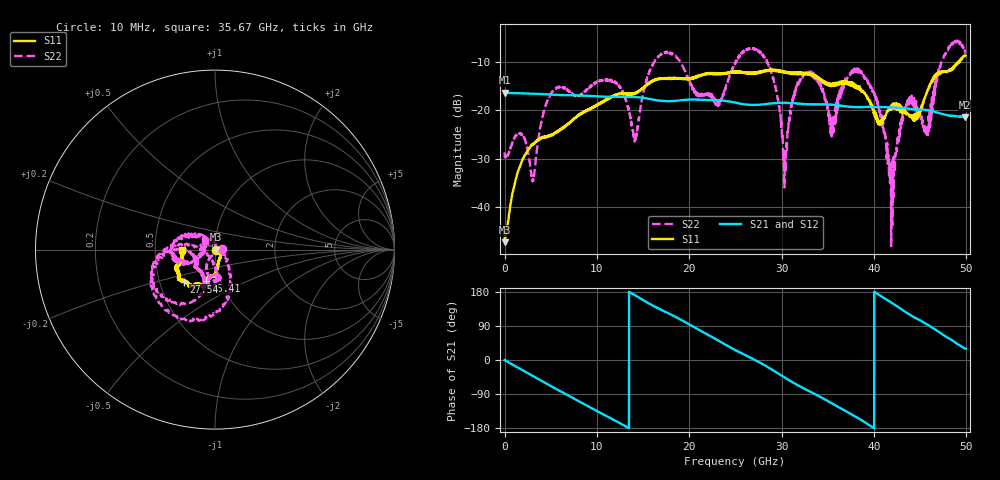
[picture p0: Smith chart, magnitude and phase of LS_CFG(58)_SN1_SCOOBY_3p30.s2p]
!Keysight Technologies,N5245B,MY58422026,A.13.80.08
!Date: Thursday, March 19, 2020 23:45:07
!Correction: S11(Full 2 Port(1,2))
!S21(Full 2 Port(1,2))
!S12(Full 2 Port(1,2))
!S22(Full 2 Port(1,2))
!S2P File: Measurements: S11, S21, S12, S22:
# Hz S DB R 50.0
!freq dBS11 angS11 dBS21 angS21 dBS12 angS12 dBS22 angS22
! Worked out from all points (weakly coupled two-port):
!   4991 points, 10 MHz to 49.91 GHz, reference 50 ohm
!   highest |S21| = -16.38 dB at 10 MHz (marker M1); lowest = -21.4 dB at 49.82 GHz (marker M2)
!   lowest |S11| = -47.2 dB at 30 MHz (marker M3), VSWR 1.01, Z = 50.4 - j0.0242 ohm
!   |S11| at or under -10 dB: start of sweep to 49.13 GHz; 49.1623 GHz to 49.22728 GHz (64.98 MHz wide, 0.132 % of centre)
!   |S22| runs from -48.0 to -5.6 dB; largest |S21 - S12| = 0.0015
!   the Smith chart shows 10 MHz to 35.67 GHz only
!   S11 on the Smith chart (normalised r, x): 10 MHz: 1.01, -0.01; 15.41 GHz: 0.85, -0.31; 27.54 GHz: 0.66, -0.25; 35.67 GHz: 0.69, -0.01
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1e7  -45.23 -31.8  -16.38 -0.3  -16.37 -0.3  -28.66 1.0
3e7  -47.24 -3.2  -16.39 -0.5  -16.37 -0.5  -29.46 -3.1
2.47e9  -28.35 -42.9  -16.54 -34.1  -16.53 -34.0  -27.83 -17.0
3.12e9  -26.99 -47.3  -16.58 -42.9  -16.57 -42.8  -34.41 -77.1
5.37e9  -24.70 -64.9  -16.79 -73.4  -16.78 -73.4  -15.79 -97.7
8.33e9  -20.75 -80.5  -16.95 -112.7  -16.95 -112.7  -16.71 -95.3
1.208e10  -16.81 -91.1  -17.23 -161.2  -17.22 -161.1  -14.25 -90.5
1.413e10  -16.48 -100.7  -17.25 170.8  -17.25 170.9  -25.74 -137.8
1.541e10  -14.81 -106.2  -17.54 152.4  -17.54 152.5  -13.72 172.9
1.665e10  -13.58 -107.1  -17.97 136.1  -17.96 136.2  -8.98 -165.3
2.312e10  -12.58 -121.3  -17.91 51.8  -17.92 52.0  -19.10 -153.7
2.496e10  -12.17 -126.1  -18.38 26.5  -18.37 26.7  -10.42 -171.0
2.754e10  -12.05 -134.2  -18.85 -5.3  -18.84 -5.1  -7.79 -104.6
3.037e10  -12.19 -145.2  -18.45 -46.7  -18.45 -46.4  -30.23 40.5
3.148e10  -12.26 -151.3  -18.54 -62.7  -18.54 -62.4  -15.58 145.8
3.328e10  -12.64 -157.7  -18.76 -86.0  -18.76 -85.7  -12.37 -168.6
3.567e10  -14.81 -178.9  -18.87 -117.3  -18.81 -116.8  -22.47 140.6
3.85e10  -15.42 175.4  -19.34 -156.5  -19.31 -156.7  -12.16 -156.7
4.16e10  -19.68 102.3  -19.38 156.0  -19.40 155.9  -30.30 73.8
4.675e10  -12.48 5.1  -20.42 79.0  -20.44 79.2  -13.58 -137.5
4.982e10  -8.77 -16.6  -21.42 30.8  -21.43 31.0  -7.42 -12.8
4.991e10  -8.71 -15.6  -21.40 29.8  -21.43 29.8  -8.05 -13.1
